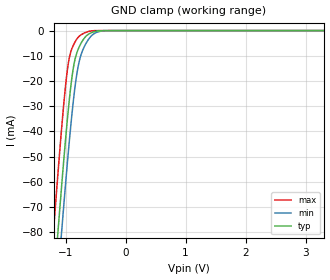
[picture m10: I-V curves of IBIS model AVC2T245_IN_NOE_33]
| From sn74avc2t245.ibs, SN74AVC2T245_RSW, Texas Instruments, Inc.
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[Model]   AVC2T245_IN_NOE_33
Model_type  Input
Vinl=0.8
Vinh=2.0
| variable   typ   min   max
C_comp   2.70pF   1.98pF   3.18pF
[Temperature Range]   40   100   -40
| Ambient temperature   25   85   -40
[Voltage range]   3.3   3   3.6
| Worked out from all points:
|   GND clamp passes 1 mA (typ) near -0.58 V on its own axis
[GND Clamp]
| AVC2T245_IN_NOE_33
|   Voltage   I(typ)   I(min)   I(max)
-4.6V     -1.266A    -1.277A    -1.254A
-1.205V   -104.2mA   -122.6mA   -80.97mA
-1.135V   -82.53mA   -100.9mA   -59.27mA
-1.115V   -76.45mA   -94.78mA   -53.25mA
-1.065V   -61.6mA    -79.78mA   -38.73mA
-955mV    -31.71mA   -48.62mA   -13.24mA
-880mV    -16.34mA   -30.09mA   -6.352mA
-810mV    -8.703mA   -16.94mA   -3.298mA
-675mV    -2.646mA   -5.774mA   -841.1uA
-540mV    -570.8uA   -1.478mA   -61.72uA
-340mV    -6.933uA   -59.19uA   -50.62nA
3.3V      193.8pA    23.09nA    42.91pA
